| TEXAS INSTRUMENTS INCORPORATED
| Standard Linear and Logic Group
| IBIS Model of TWL1200
| SDIO, UART, AND AUDIO VOLTAGE-TRANSLATION TRANSCEIVER
| This file contains package information for the following:
|  BGA 48-pin (ZQC) package as [Component] TWL1200_ZQC
| (See IBIS file twl1200_yff.ibs for WCSP-YFF package information as
|  simulation die data is different)
| This device can be powered at the following Vccs:
|  3.3 volt Vcc
|  2.5 volt Vcc
|  1.8 volt Vcc
|  1.5 volt Vcc
|  1.2 volt Vcc
| This file provides unique models under the [Model Selector] for each Vcc.
| For operation at a specific Vcc, select the appropriate model after each
| [Model Selector] keyword.
[IBIS Ver]   3.2
[Comment char]  |_char
[File Name]   twl1200_zqc.ibs
[File Rev]   1.1 | X
[Date]   January 13, 2010
[Source]   Data created from TI-SPICE simulations at TI-SLL.
[Notes]   The following is an IBIS list for the TWL1200.
   Please contact sllibis@ti.com with questions and
   comments concerning SLL IBIS models.
   Note: The IOASDA & IOASDB have a model selector to show the
   different drive levels of the circuit.  The non-_DC model
   demonstrates the full drive circuit used for voltage
   transitions, and the _DC model represents the weaker/low-power
   drive circuit for holding DC levels.
   - FILE REV HISTORY
   - 1.1 Release IBIS file on 1/14/2010
   - Power clamp data deleted was deleted as there is no
   power-clamp diode.
[Disclaimer]
 This model is designed as an aid for customers of Texas Instruments.
 TI and its licensors and suppliers make no warranties, either expressed
 or implied, with respect to this  model, including the warranties of
 merchantability or fitness for a particular purpose.
 The model is provided solely on an "as is" basis. The entire risk as to
 its quality and performance is with the customer.
[Copyright] (C)Copyright 2009 Texas Instruments Incorporated.
   All rights reserved.
| Component TWL1200_ZQC 48-PIN JRBGA
[Component]   TWL1200_ZQC
[Manufacturer]   Texas Instruments, Inc.
[Package]
|   typ   min   max
R_pkg   5.800e-02   4.500e-02   8.300e-02
L_pkg   1.425e-09   1.108e-09   2.187e-09
C_pkg   1.560e-13   1.290e-13   2.290e-13
[Pin]   signal_name   model_name   R_pin   L_pin   C_pin
A1   SDIO_CLK_A AIN   4.600e-02   1.138e-09   1.330e-13
A2   SDIO_CMD_A IOASDA   4.500e-02   1.108e-09   1.300e-13
A3   AUDIO_CLK_A AIO_4MA   5.900e-02   1.453e-09   1.640e-13
A4   AUD_DIR   CONTROLIN   6.600e-02   1.633e-09   1.620e-13
A5   AUDIO_CLK_B BIO_4MA   4.500e-02   1.108e-09   1.300e-13
A6   SDIO_CMD_B IOASDB   7.200e-02   1.787e-09   1.970e-13
A7   SDIO_CLK_B BOUT_8MA   6.100e-02   1.508e-09   1.700e-13
B1   SDIO_DATA3_A IOASDA   5.900e-02   1.451e-09   1.650e-13
B2   SDIO_DATA0_A IOASDA   5.000e-02   1.220e-09   1.400e-13
B3   AUDIO_FSYNC_A AOUT_4MA   4.500e-02   1.108e-09   1.300e-13
B4   OE   CONTROLIN   5.000e-02   1.223e-09   1.390e-13
B5   AUDIO_FSYNC_B BIN   6.600e-02   1.631e-09   1.630e-13
B6   SDIO_DATA0_B IOASDB   7.200e-02   1.796e-09   1.970e-13
B7   SDIO_DATA3_B IOASDB   5.000e-02   1.222e-09   1.390e-13
C1   SDIO_DATA2_A IOASDA   4.600e-02   1.137e-09   1.330e-13
C2   SDIO_DATA1_A IOASDA   6.100e-02   1.508e-09   1.690e-13
C4   VCCA   POWER   5.700e-02   1.376e-09   1.290e-13
C5   VCCB   POWER   4.600e-02   1.137e-09   1.330e-13
C6   SDIO_DATA1_B IOASDB   4.600e-02   1.138e-09   1.330e-13
C7   SDIO_DATA2_B IOASDB   6.100e-02   1.508e-09   1.690e-13
D1   WLAN_EN_A  AIN   5.000e-02   1.220e-09   1.400e-13
D2   WLAN_IRQ_A AOUT_4MA   4.500e-02   1.108e-09   1.300e-13
D3   GND   GND   5.700e-02   1.375e-09   1.310e-13
D4   VCCA   POWER   8.300e-02   2.187e-09   2.290e-13
D5   VCCB   POWER   5.900e-02   1.452e-09   1.640e-13
D6   WLAN_EN_B  BOUT_2MA   6.100e-02   1.509e-09   1.690e-13
D7   WLAN_IRQ_B BIN   7.300e-02   1.810e-09   1.980e-13
E1   CLK_REQ_A  AOUT_8MA   5.700e-02   1.376e-09   1.290e-13
E2   BT_EN_A   AIN   7.200e-02   1.790e-09   1.960e-13
E3   GND   GND   7.800e-02   1.918e-09   1.980e-13
E4   GND   GND   5.000e-02   1.220e-09   1.400e-13
E5   GND   GND   6.100e-02   1.508e-09   1.690e-13
E6   BT_EN_B   BOUT_4MA   4.600e-02   1.138e-09   1.320e-13
E7   CLK_REQ_B  BIN   7.900e-02   1.954e-09   1.980e-13
F1   BT_UART_CTS_A AIN   5.000e-02   1.220e-09   1.390e-13
F2   BT_UART_RTS_A AOUT_4MA   5.000e-02   1.223e-09   1.380e-13
F3   AUDIO_IN_A AIN   6.100e-02   1.509e-09   1.690e-13
F4   SLOW_CLK_B BOUT_2MA   6.100e-02   1.507e-09   1.690e-13
F5   AUDIO_IN_B BOUT_4MA   4.600e-02   1.138e-09   1.320e-13
F6   BT_UART_RTS_B BIN   6.600e-02   1.632e-09   1.560e-13
F7   BT_UART_CTS_B BOUT_4MA   6.100e-02   1.508e-09   1.690e-13
G1   BT_UART_RX_A AIN   5.000e-02   1.223e-09   1.390e-13
G2   BT_UART_TX_A AOUT_8MA   4.600e-02   1.137e-09   1.330e-13
G3   AUD_OUT_A  AOUT_4MA   5.700e-02   1.376e-09   1.290e-13
G4   SLOW_CLK_A AIN   4.600e-02   1.138e-09   1.330e-13
G5   AUD_OUT_B  BIN   7.900e-02   1.968e-09   2.000e-13
G6   BT_UART_TX_B BIN   5.900e-02   1.453e-09   1.640e-13
G7   BT_UART_RX_B BOUT_8MA   6.600e-02   1.632e-09   1.620e-13
| Model BIO_4MA
[Model Selector]   BIO_4MA
BIO_4MA_33   3.3 volt Vcc
BIO_4MA_25   2.5 volt Vcc
BIO_4MA_18   1.8 volt Vcc
BIO_4MA_15A   1.5 volt Vcc
BIO_4MA_12   1.2 volt Vcc
| Model CONTROLIN
[Model Selector]   CONTROLIN
CONTROLIN_33   3.3 volt Vcc
CONTROLIN_25   2.5 volt Vcc
CONTROLIN_18   1.8 volt Vcc
CONTROLIN_15A   1.5 volt Vcc
CONTROLIN_12   1.2 volt Vcc
| Model AIN
[Model Selector]   AIN
AIN_33   3.3 volt Vcc
AIN_25   2.5 volt Vcc
AIN_18   1.8 volt Vcc
AIN_15A   1.5 volt Vcc
AIN_12   1.2 volt Vcc
| Model BIN
[Model Selector]   BIN
BIN_33   3.3 volt Vcc
BIN_25   2.5 volt Vcc
BIN_18   1.8 volt Vcc
BIN_15A   1.5 volt Vcc
BIN_12   1.2 volt Vcc
| Model IOASDB
[Model Selector]   IOASDB
IOASDB_33   3.3 volt Vcc
IOASDB_25   2.5 volt Vcc
IOASDB_18   1.8 volt Vcc
IOASDB_15A   1.5 volt Vcc
IOASDB_12   1.2 volt Vcc
| Model IOASDA_DC
[Model Selector]   IOASDA_DC
IOASDA_DC_33   3.3 volt Vcc
IOASDA_DC_25   2.5 volt Vcc
IOASDA_DC_18   1.8 volt Vcc
IOASDA_DC_15A   1.5 volt Vcc
IOASDA_DC_12   1.2 volt Vcc
| Model IOASDA
[Model Selector]   IOASDA
IOASDA_33   3.3 volt Vcc
IOASDA_25   2.5 volt Vcc
IOASDA_18   1.8 volt Vcc
IOASDA_15A   1.5 volt Vcc
IOASDA_12   1.2 volt Vcc
| Model IOASDB_DC
[Model Selector]   IOASDB_DC
IOASDB_DC_33   3.3 volt Vcc
IOASDB_DC_25   2.5 volt Vcc
IOASDB_DC_18   1.8 volt Vcc
IOASDB_DC_15A   1.5 volt Vcc
IOASDB_DC_12   1.2 volt Vcc
| Model BOUT_8MA
[Model Selector]   BOUT_8MA
BOUT_8MA_33   3.3 volt Vcc
BOUT_8MA_25   2.5 volt Vcc
BOUT_8MA_18   1.8 volt Vcc
BOUT_8MA_15A   1.5 volt Vcc
BOUT_8MA_12   1.2 volt Vcc
| Model AIO_4MA
[Model Selector]   AIO_4MA
AIO_4MA_33   3.3 volt Vcc
AIO_4MA_25   2.5 volt Vcc
AIO_4MA_18   1.8 volt Vcc
AIO_4MA_15A   1.5 volt Vcc
AIO_4MA_12   1.2 volt Vcc
| Model AOUT_8MA
[Model Selector]   AOUT_8MA
AOUT_8MA_33   3.3 volt Vcc
AOUT_8MA_25   2.5 volt Vcc
AOUT_8MA_18   1.8 volt Vcc
AOUT_8MA_15A   1.5 volt Vcc
AOUT_8MA_12   1.2 volt Vcc
| Model AOUT_4MA
[Model Selector]   AOUT_4MA
AOUT_4MA_33   3.3 volt Vcc
AOUT_4MA_25   2.5 volt Vcc
AOUT_4MA_18   1.8 volt Vcc
AOUT_4MA_15A   1.5 volt Vcc
AOUT_4MA_12   1.2 volt Vcc
| Model BOUT_4MA
[Model Selector]   BOUT_4MA
BOUT_4MA_33   3.3 volt Vcc
BOUT_4MA_25   2.5 volt Vcc
BOUT_4MA_18   1.8 volt Vcc
BOUT_4MA_15A   1.5 volt Vcc
BOUT_4MA_12   1.2 volt Vcc
| Model BOUT_2MA
[Model Selector]   BOUT_2MA
BOUT_2MA_33   3.3 volt Vcc
BOUT_2MA_25   2.5 volt Vcc
BOUT_2MA_18   1.8 volt Vcc
BOUT_2MA_15A   1.5 volt Vcc
BOUT_2MA_12   1.2 volt Vcc
| Models and submodels in the file (70): BIO_4MA_33 (Input), BIO_4MA_25 (Input), BIO_4MA_18 (Input), BIO_4MA_15A (Input), BIO_4MA_12 (Input), CONTROLIN_33 (Input), CONTROLIN_25 (Input), CONTROLIN_18 (Input), CONTROLIN_15A (Input), CONTROLIN_12 (Input), AIN_33 (Input), AIN_25 (Input), AIN_18 (Input), AIN_15A (Input), AIN_12 (Input), BIN_33 (Input), BIN_25 (Input), BIN_18 (Input), BIN_15A (Input), BIN_12 (Input), IOASDB_33 (I/O), IOASDB_25 (I/O), IOASDB_18 (I/O), IOASDB_15A (I/O), IOASDB_12 (I/O), IOASDA_DC_33 (I/O), IOASDA_DC_25 (I/O), IOASDA_DC_18 (I/O), IOASDA_DC_15A (I/O), IOASDA_DC_12 (I/O), IOASDA_33 (I/O), IOASDA_25 (I/O), IOASDA_18 (I/O), IOASDA_15A (I/O), IOASDA_12 (I/O), IOASDB_DC_33 (I/O), IOASDB_DC_25 (I/O), IOASDB_DC_18 (I/O), IOASDB_DC_15A (I/O), IOASDB_DC_12 (I/O), BOUT_8MA_33 (Output), BOUT_8MA_25 (Output), BOUT_8MA_18 (Output), BOUT_8MA_15A (Output), BOUT_8MA_12 (Output), AIO_4MA_33 (Output), AIO_4MA_25 (Output), AIO_4MA_18 (Output), AIO_4MA_15A (Output), AIO_4MA_12 (Output), AOUT_8MA_33 (Output), AOUT_8MA_25 (Output), AOUT_8MA_18 (Output), AOUT_8MA_15A (Output), AOUT_8MA_12 (Output), AOUT_4MA_33 (Output), AOUT_4MA_25 (Output), AOUT_4MA_18 (Output), AOUT_4MA_15A (Output), AOUT_4MA_12 (Output), BOUT_4MA_33 (Output), BOUT_4MA_25 (Output), BOUT_4MA_18 (Output), BOUT_4MA_15A (Output), BOUT_4MA_12 (Output), BOUT_2MA_33 (Output), BOUT_2MA_25 (Output), BOUT_2MA_18 (Output), BOUT_2MA_15A (Output), BOUT_2MA_12 (Output)
